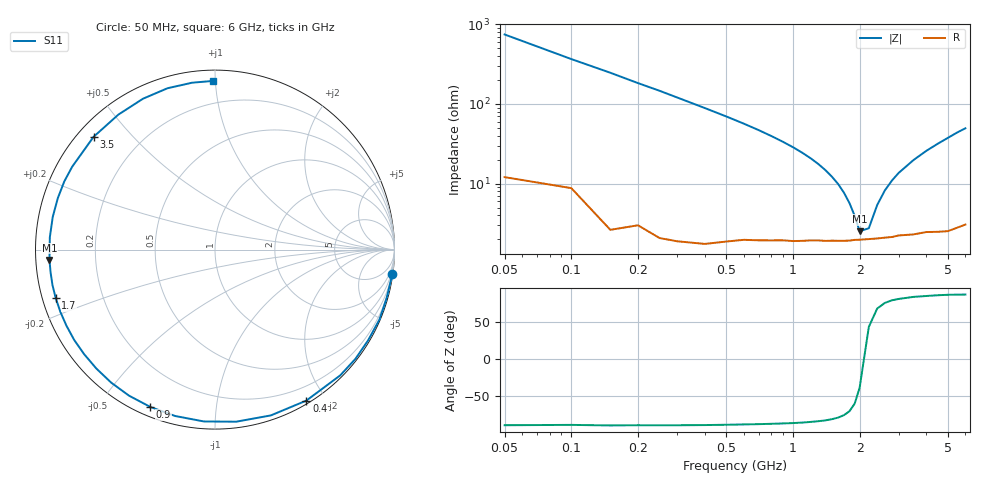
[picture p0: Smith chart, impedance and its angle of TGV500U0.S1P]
! SIEMENS Discrete & RF Semiconductors
! BAT64
! Si Schottky Diode in SOT23
! VR = 0.5 V
! S-Parameters:  February  1997
# GHz  S  MA  R  50
!  f  S11
! GHz  MAG  ANG
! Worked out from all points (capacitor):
!   34 points, 50 MHz to 6 GHz, reference 50 ohm
!   read as one part to ground: C = 4.3 pF near 50 MHz
!   lowest |Z| = 2.52 ohm at 2 GHz (marker M1)
!   series resonance near 2.091 GHz, so ESL is about 1.3 nH
!   S11 on the Smith chart (normalised r, x): 50 MHz: 0, -15; 400 MHz: 0.03, -1.77; 900 MHz: 0.04, -0.67; 1.7 GHz: 0.04, -0.15; 3.5 GHz: 0.05, +0.39; 6 GHz: 0.06, +0.99
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0.05  0.9978 -7.7
0.15  0.9958 -23.0
0.2  0.9916 -30.7
0.25  0.9913 -37.8
0.3  0.9889 -45.1
0.4  0.9833 -58.8
0.5  0.9748 -71.4
0.6  0.966 -83.0
0.7  0.9595 -93.7
0.8  0.9533 -103.5
0.9  0.9478 -112.4
1  0.9443 -120.5
1.1  0.9401 -128.0
1.2  0.936 -134.9
1.4  0.9321 -147.3
1.6  0.9288 -158.1
1.7  0.9277 -163.1
2  0.9241 -176.4
2.2  0.9228 175.7
2.4  0.9221 168.6
2.6  0.9215 161.9
3  0.9201 149.9
3.5  0.9233 137.1
4  0.9249 125.6
4.5  0.9315 115.5
5  0.9372 106.4
5.5  0.9386 97.8
6  0.9398 90.7
